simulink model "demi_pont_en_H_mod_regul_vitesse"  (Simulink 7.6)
settings: Solver=ode15s  StartTime=0.0  StopTime=2  RelTol=1e-3
InitFcn:
  | clc
  | delete *.mat
  | clear all
  | 
  | clc
  | 
  | Ti=0.01;
  | Kp=0.5;
  | 
  | R1=1e3;
  | R2=Kp*R1;
  | 
  | R=10e3;
  | C= Ti/R;
StopFcn:
  | close all, clc
  | load regul_vitesse.mat
  | plot(x(1,:),x(2,:),x(1,:),x(4,:))
  | 
  | 
  | xlabel('temps')
  | axis([0 2 -100 3000])
  | title('Position et vitesse angulaires - Moteur CC, 1/2 Pont en H')
  | grid
undefined symbols (not defined in the file or in its folder): sigbuilder_block
libraries: fl_lib x12, elec_lib x10, nesl_utility x4

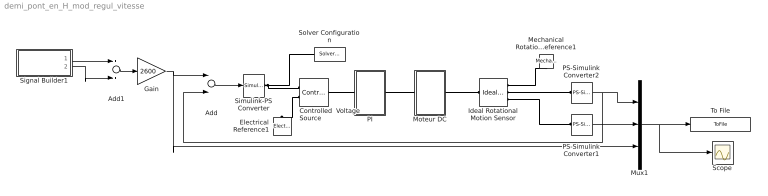
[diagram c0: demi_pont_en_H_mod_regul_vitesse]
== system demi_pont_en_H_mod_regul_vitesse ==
  Add : Sum  Inputs=+-
  Add1 : Sum
  Controlled  Voltage Source : fl_lib/Electrical/Electrical Sources/Controlled Voltage Source  DialogController=NetworkEngine.DynNeDlgSource  SystemSampleTime=-1  i_Log=off  v_Log=off  LocalVarNames=|i|v  LocalVarDescs=|i|v  LocalVarLogging=[0 0]
  Electrical Reference1 : fl_lib/Electrical/Electrical Elements/Electrical Reference  DialogController=NetworkEngine.DynNeDlgSource  SystemSampleTime=-1  i_Log=off  LocalVarNames=|i  LocalVarDescs=|i  LocalVarLogging=[]
  Gain : Gain  Gain=2600
  Ideal Rotational Motion Sensor : fl_lib/Mechanical/Mechanical Sensors/Ideal Rotational Motion Sensor  DialogController=NetworkEngine.DynNeDlgSource  SystemSampleTime=-1  offset=0 rad  w_Log=off  t_Log=off  phi_Log=off  LocalVarNames=|w|t|phi  LocalVarDescs=|w|t|phi  LocalVarLogging=[0 0 0]
  Mechanical Rotational Reference1 : fl_lib/Mechanical/Rotational Elements/Mechanical Rotational Reference  DialogController=NetworkEngine.DynNeDlgSource  SystemSampleTime=-1  t_Log=off  LocalVarNames=|t  LocalVarDescs=|t  LocalVarLogging=0
  Moteur DC : Subsystem
  Mux1 : Mux  Inputs=3
  PI : Subsystem
  PS-Simulink Converter1 : nesl_utility/PS-Simulink Converter  DialogController=NetworkEngine.DynNeUtilDlgSource  SystemSampleTime=-1  PhysicalDomain=network_engine_domain  LeftPortType=input  RightPortType=output  SubClassName=ps_output  Unit=1  AffineConversion=off
  PS-Simulink Converter2 : nesl_utility/PS-Simulink Converter  DialogController=NetworkEngine.DynNeUtilDlgSource  SystemSampleTime=-1  PhysicalDomain=network_engine_domain  LeftPortType=input  RightPortType=output  SubClassName=ps_output  Unit=1  AffineConversion=off
  Scope : Scope
  Signal Builder1 : Subsystem  Tag=STV Subsys  LoadFcn=sigbuilder_block('load');  StartFcn=sigbuilder_block('start');  StopFcn=sigbuilder_block('stop');  ClipboardFcn=sigbuilder_block('clipboard');
  Simulink-PS Converter : nesl_utility/Simulink-PS Converter  DialogController=NetworkEngine.DynNeUtilDlgSource  SystemSampleTime=-1  PhysicalDomain=network_engine_domain  LeftPortType=input  RightPortType=output  SubClassName=ps_input  Unit=1  AffineConversion=off  InputFilterTimeConstant=.001  UdotUserProvided=0
  Solver Configuration : nesl_utility/Solver Configuration  DialogController=NetworkEngine.DynNeUtilDlgSource  SystemSampleTime=-1  PhysicalDomain=network_engine_domain  LeftPortType=input  RightPortType=generic  SubClassName=solver  Accelerate=off  Profile=off  ResidualTolerance=1e-9  MaxNonlinIter=12  MaxModeIter=2  DoFixedCost=off  UseLocalSampling=off  DoDC=off  LinearAlgebra=Sparse  LocalSolverSampleTime=.001  LocalSolverChoice=NE_BACKWARD_EULER_ADVANCER  UseLocalSolver=off
  To File : ToFile  Filename=regul_vitesse  MatrixName=x
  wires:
  PS-Simulink Converter1/1 -> Mux1/2
  PS-Simulink Converter2/1 -> Mux1/1, Add/2
  Mux1/1 -> Scope/1, To File/1
  Add/1 -> Simulink-PS Converter/1
  Gain/1 -> Add/1, Mux1/3
  Add1/1 -> Gain/1
  Signal Builder1/1(Signal 1) -> Add1/1
  Signal Builder1/2(Signal 2) -> Add1/2
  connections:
  Simulink-PS Converter/RConn1 -- Controlled  Voltage Source/RConn1 -- Solver Configuration/RConn1
  Ideal Rotational Motion Sensor/LConn1 -- Moteur DC/RConn1
  Controlled  Voltage Source/RConn2 -- Electrical Reference1/LConn1
  Ideal Rotational Motion Sensor/RConn3 -- PS-Simulink Converter1/LConn1
  Ideal Rotational Motion Sensor/RConn2 -- PS-Simulink Converter2/LConn1
  Ideal Rotational Motion Sensor/RConn1 -- Mechanical Rotational Reference1/LConn1
  PI/RConn1 -- Moteur DC/LConn1
  Controlled  Voltage Source/LConn1 -- PI/LConn1

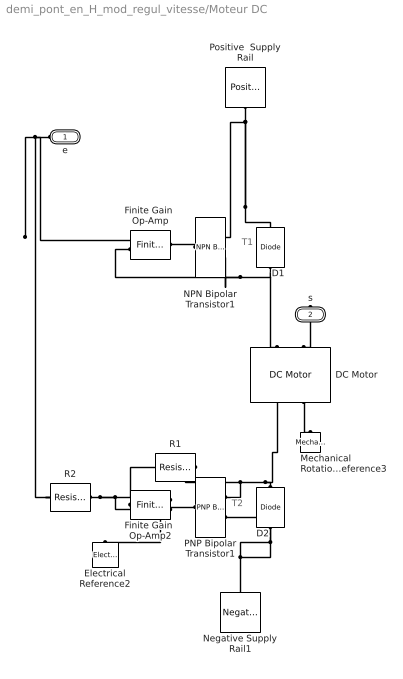
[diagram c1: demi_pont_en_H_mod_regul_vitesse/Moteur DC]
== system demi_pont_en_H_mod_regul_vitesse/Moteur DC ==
  note: T1
  note: T2
  D1 : elec_lib/Semiconductor Devices/Diode  DialogController=NetworkEngine.DynNeDlgSource  SystemSampleTime=-1  ModelType=1  Vf=0.6 V  Ron=0.3 Ohm  Goff=1e-8 S  Rz=0.3 Ohm  Vz=50 V  C_PWL=5 pF  prmExp=1  I12=[ 0.07 1.5 ] A  V12=[ 0.7 0.8 ] V  I1=0.07 A  V1=0.7 V  RS=0.01 Ohm  IS=1e-14 A  Tmeas=25 C  ec=1  BV=Inf V  C_param=1  CJ0=5 pF  VJ=1 V  Mgrad=0.5  Vvec=[ 0.1 10 100 ] V  Cvec=[ 3.5 1 0.4 ] pF  FC=0.5  LocalVarLogging=[]
  D2 : elec_lib/Semiconductor Devices/Diode  DialogController=NetworkEngine.DynNeDlgSource  SystemSampleTime=-1  ModelType=1  Vf=0.6 V  Ron=0.3 Ohm  Goff=1e-8 S  Rz=0.3 Ohm  Vz=50 V  C_PWL=5 pF  prmExp=1  I12=[ 0.07 1.5 ] A  V12=[ 0.7 0.8 ] V  I1=0.07 A  V1=0.7 V  RS=0.01 Ohm  IS=1e-14 A  Tmeas=25 C  ec=1  BV=Inf V  C_param=1  CJ0=5 pF  VJ=1 V  Mgrad=0.5  Vvec=[ 0.1 10 100 ] V  Cvec=[ 3.5 1 0.4 ] pF  FC=0.5  LocalVarLogging=[]
  DC Motor : elec_lib/Actuators & Drivers/Rotational Actuators/DC Motor  DialogController=NetworkEngine.DynNeDlgSource  SystemSampleTime=-1  parameterization=1  Ra=3.9 Ohm  La=1.2e-5 H  emf_or_torque=1  Kv=7.2e-5 V/rpm  Ki=6.876e-4 N*m/A  T_stall=2.4e-4 N*m  w_max=1.91e+4 rpm  w_rated=1.5e+4 rpm  P_rated=0.08 W  V_rated=1.5 V  J=0.01 g*cm^2  lam=1e-8 N*m/(rad/s)  speed0=0.5 rpm  current_Log=off  voltage_Log=off  power_Log=off  i2r_Log=off  torque_Log=off  speed_Log=off  LocalVarNames=|current|voltage|power|i2r|torque|speed  LocalVarDescs=|Current (A)|Voltage (V)|Power (W)|Electrical losses (W)|Torque (Nm)|Angular speed (rad/s)  LocalVarLogging=[0 0 0 0 0 0]
  Electrical Reference2 : fl_lib/Electrical/Electrical Elements/Electrical Reference  DialogController=NetworkEngine.DynNeDlgSource  SystemSampleTime=-1  i_Log=off  LocalVarNames=|i  LocalVarDescs=|i  LocalVarLogging=[]
  Finite Gain  Op-Amp : elec_lib/Integrated Circuits/Finite Gain Op-Amp  DialogController=NetworkEngine.DynNeDlgSource  SystemSampleTime=-1  A=1000  Rin=1e+6 Ohm  Rout=100 Ohm  Vmin=-15 V  Vmax=15 V  LocalVarLogging=[]
  Finite Gain  Op-Amp2 : elec_lib/Integrated Circuits/Finite Gain Op-Amp  DialogController=NetworkEngine.DynNeDlgSource  SystemSampleTime=-1  A=1000  Rin=1e+6 Ohm  Rout=100 Ohm  Vmin=-15 V  Vmax=15 V  LocalVarLogging=[]
  Mechanical Rotational Reference3 : fl_lib/Mechanical/Rotational Elements/Mechanical Rotational Reference  DialogController=NetworkEngine.DynNeDlgSource  SystemSampleTime=-1  t_Log=off  LocalVarNames=|t  LocalVarDescs=|t  LocalVarLogging=0
  NPN Bipolar Transistor1 : elec_lib/Semiconductor Devices/NPN Bipolar Transistor  DialogController=NetworkEngine.DynNeDlgSource  SystemSampleTime=-1  parameterization=1  BF=100  IS=1e-14 A  VAF=200 V  hfe=100  hoe=5e-5 1/Ohm  Ic_h=1 mA  V1=0.55 V  I1=0.5 mA  BR=1  Tmeas=25 C  RC=0.01 Ohm  RE=1e-4 Ohm  RB=1 Ohm  C_BC=5 pF  C_BE=5 pF  TF=0 us  TR=0 us  LocalVarLogging=[]
  Negative Supply Rail1 : elec_lib/Sources/Negative Supply Rail  DialogController=NetworkEngine.DynNeDlgSource  SystemSampleTime=-1  v0=-24 V  current_Log=off  voltage_Log=off  power_Log=off  LocalVarNames=|current|voltage|power  LocalVarDescs=|Current (A)|Voltage (V)|Power (W)  LocalVarLogging=[0 0 0]
  PNP Bipolar Transistor1 : elec_lib/Semiconductor Devices/PNP Bipolar Transistor  DialogController=NetworkEngine.DynNeDlgSource  SystemSampleTime=-1  parameterization=1  BF=100  IS=1e-14 A  VAF=200 V  hfe=100  hoe=5e-5 1/Ohm  Ic_h=1 mA  V1=0.55 V  I1=0.5 mA  BR=1  Tmeas=25 C  RC=0.01 Ohm  RE=1e-4 Ohm  RB=1 Ohm  C_BC=5 pF  C_BE=5 pF  TF=0 us  TR=0 us  LocalVarLogging=[]
  Positive  Supply Rail : elec_lib/Sources/Positive Supply Rail  DialogController=NetworkEngine.DynNeDlgSource  SystemSampleTime=-1  v0=24 V  current_Log=off  voltage_Log=off  power_Log=off  LocalVarNames=|current|voltage|power  LocalVarDescs=|Current (A)|Voltage (V)|Power (W)  LocalVarLogging=[0 0 0]
  R1 : fl_lib/Electrical/Electrical Elements/Resistor  DialogController=NetworkEngine.DynNeDlgSource  SystemSampleTime=-1  R=10 kOhm  i_Log=off  v_Log=off  LocalVarNames=|i|v  LocalVarDescs=|i|v  LocalVarLogging=[0 0]
  R2 : fl_lib/Electrical/Electrical Elements/Resistor  DialogController=NetworkEngine.DynNeDlgSource  SystemSampleTime=-1  R=10 kOhm  i_Log=off  v_Log=off  LocalVarNames=|i|v  LocalVarDescs=|i|v  LocalVarLogging=[0 0]
  e : PMIOPort  Port=1  Side=Left
  s : PMIOPort  Port=2  Side=Right
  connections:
  D1/LConn1 -- Finite Gain  Op-Amp/LConn2 -- NPN Bipolar Transistor1/RConn2 -- DC Motor/LConn1
  Positive  Supply Rail/RConn1 -- NPN Bipolar Transistor1/RConn1 -- D1/RConn1
  D2/LConn1 -- Negative Supply Rail1/LConn1 -- PNP Bipolar Transistor1/RConn2
  D2/RConn1 -- DC Motor/RConn1 -- R1/RConn1 -- PNP Bipolar Transistor1/RConn1
  DC Motor/RConn2 -- Mechanical Rotational Reference3/LConn1
  Finite Gain  Op-Amp2/LConn1 -- Electrical Reference2/LConn1
  e/RConn1 -- Finite Gain  Op-Amp/LConn1 -- R2/LConn1
  NPN Bipolar Transistor1/LConn1 -- Finite Gain  Op-Amp/RConn1
  Finite Gain  Op-Amp2/LConn2 -- R2/RConn1 -- R1/LConn1
  Finite Gain  Op-Amp2/RConn1 -- PNP Bipolar Transistor1/LConn1
  s/RConn1 -- DC Motor/LConn2

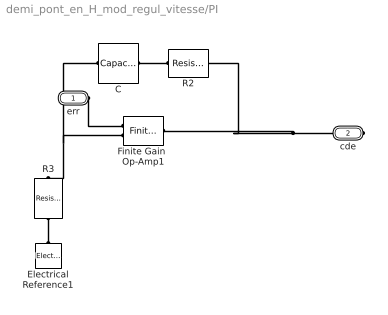
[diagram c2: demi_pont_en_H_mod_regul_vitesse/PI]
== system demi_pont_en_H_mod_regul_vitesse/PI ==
  C : fl_lib/Electrical/Electrical Elements/Capacitor  DialogController=NetworkEngine.DynNeDlgSource  SystemSampleTime=-1  c=C F  v0=0 V  r=1e-6 Ohm  g=0 1/Ohm  i_Log=off  v_Log=off  vc_Log=off  LocalVarNames=|i|v|vc  LocalVarDescs=|i|v|Internal variable for voltage across capacitor term  LocalVarLogging=[0 0 0]
  Electrical Reference1 : fl_lib/Electrical/Electrical Elements/Electrical Reference  DialogController=NetworkEngine.DynNeDlgSource  SystemSampleTime=-1  i_Log=off  LocalVarNames=|i  LocalVarDescs=|i  LocalVarLogging=[]
  Finite Gain  Op-Amp1 : elec_lib/Integrated Circuits/Finite Gain Op-Amp  DialogController=NetworkEngine.DynNeDlgSource  SystemSampleTime=-1  A=1000  Rin=1e+6 Ohm  Rout=100 Ohm  Vmin=-15 V  Vmax=15 V  LocalVarLogging=[]
  R2 : fl_lib/Electrical/Electrical Elements/Resistor  DialogController=NetworkEngine.DynNeDlgSource  SystemSampleTime=-1  R=R Ohm  i_Log=off  v_Log=off  LocalVarNames=|current|voltage|power  LocalVarDescs=|Resistor current (A)|Voltage across resistor (V)|Power (W)  LocalVarLogging=[0 0 0]
  R3 : fl_lib/Electrical/Electrical Elements/Resistor  DialogController=NetworkEngine.DynNeDlgSource  SystemSampleTime=-1  R=R Ohm  i_Log=off  v_Log=off  LocalVarNames=|current|voltage|power  LocalVarDescs=|Resistor current (A)|Voltage across resistor (V)|Power (W)  LocalVarLogging=[0 0 0]
  err : PMIOPort  Port=1  Side=Left
  cde : PMIOPort  Port=2  Side=Right
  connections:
  C/LConn1 -- R3/RConn1 -- Finite Gain  Op-Amp1/LConn2
  C/RConn1 -- R2/LConn1
  R3/LConn1 -- Electrical Reference1/LConn1
  err/RConn1 -- Finite Gain  Op-Amp1/LConn1
  cde/RConn1 -- R2/RConn1 -- Finite Gain  Op-Amp1/RConn1

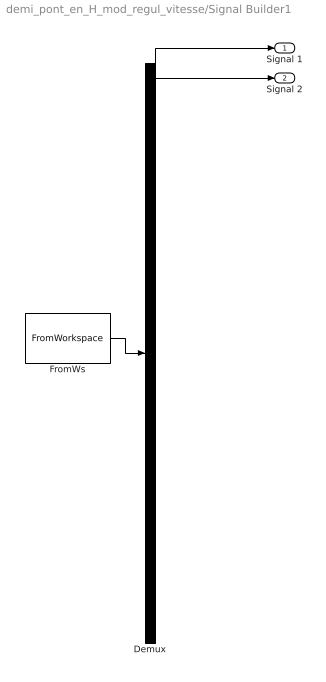
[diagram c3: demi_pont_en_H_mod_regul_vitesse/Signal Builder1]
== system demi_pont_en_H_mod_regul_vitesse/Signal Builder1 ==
  Demux : Demux  Tag=STV Demux  Outputs=2
  FromWs : FromWorkspace  Tag=STV FromWs  VariableName=tuvar  SampleTime=0  SigBuilderData=DataTag0  VnvData=DataTag1
  Signal 1 : Outport  Tag=STV Outport
  Signal 2 : Outport  Tag=STV Outport  Port=2
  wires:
  FromWs/1 -> Demux/1
  Demux/1 -> Signal 1/1
  Demux/2 -> Signal 2/1
